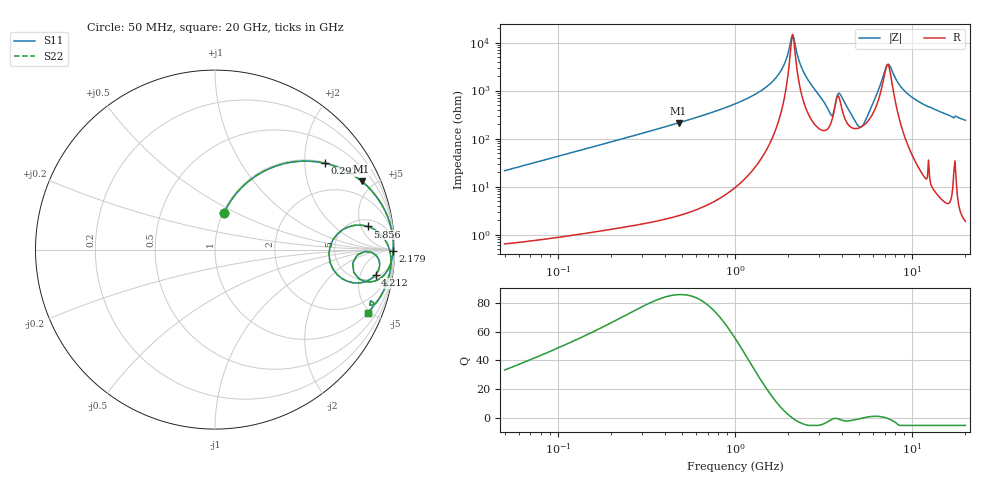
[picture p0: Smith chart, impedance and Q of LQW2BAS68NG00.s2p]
!Murata Part Number: LQW2BAS68NG00
!These Parameters are Measured in Series Mode Connection
!  o--[Z]--o
!Port1  Port2
!  o-------o
!Freq. Start=50[MHz] Stop=20[GHz], 401[Steps]
# Hz S RI R 50
!Freq.(Hz) S11(Real) S11(Imag) S21(Real) S21(Imag) S12(Real) S12(Imag) S22(Real) S22(Imag)
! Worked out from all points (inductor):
!   401 points, 50 MHz to 20 GHz, reference 50 ohm
!   read as one part in series: L = 68.3 nH near 51.52 MHz
!   highest Q = 85.5 at 480 MHz (marker M1), where L = 70.6 nH
!   self-resonance near 2.115 GHz
!   S11 on the Smith chart (normalised r, x): 50 MHz: 1.01, +0.43; 292.8 MHz: 1.03, +2.53; 2.179 GHz: open; 4.212 GHz: 6, -9; 5.856 GHz: 6.67, +6.62; 20 GHz: 1.04, -4.82
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5e7  0.0498 0.2031  0.9502 -0.2031  0.9502 -0.2031  0.0498 0.2031
1.364002e8  0.258 0.4287  0.742 -0.4287  0.742 -0.4287  0.258 0.4287
2.928045e8  0.6135 0.4805  0.3865 -0.4805  0.3865 -0.4805  0.6135 0.4805
3.721004e8  0.722 0.442  0.278 -0.442  0.278 -0.442  0.722 0.442
4.800071e8  0.8164 0.3813  0.1836 -0.3813  0.1836 -0.3813  0.8164 0.3813
1e9  0.9624 0.1814  0.0376 -0.1814  0.0376 -0.1814  0.9624 0.1814
1.639343e9  0.9917 0.0622  0.00833 -0.0622  0.00833 -0.0622  0.9917 0.0622
1.875929e9  0.9937 0.0302  0.00628 -0.0302  0.00628 -0.0302  0.9937 0.0302
2.083303e9  0.9935 0.00426  0.00654 -0.00426  0.00654 -0.00426  0.9935 0.00426
2.179053e9  0.9927 -0.00737  0.00726 0.00737  0.00726 0.00737  0.9927 -0.00737
2.383959e9  0.9899 -0.0321  0.0101 0.0321  0.0101 0.0321  0.9899 -0.0321
2.728004e9  0.9793 -0.076  0.0207 0.076  0.0207 0.076  0.9793 -0.076
3.466789e9  0.8025 -0.1628  0.1975 0.1628  0.1975 0.1628  0.8025 -0.1628
3.850025e9  0.9086 -0.0475  0.0914 0.0475  0.0914 0.0475  0.9086 -0.0475
4.212059e9  0.8949 -0.1404  0.1051 0.1404  0.1051 0.1404  0.8949 -0.1404
5.041459e9  0.6407 -0.0701  0.3593 0.0701  0.3593 0.0701  0.6407 -0.0701
5.856089e9  0.8506 0.1291  0.1494 -0.1291  0.1494 -0.1291  0.8506 0.1291
7.114996e9  0.969 0.0087  0.031 -0.0087  0.031 -0.0087  0.969 0.0087
7.442007e9  0.9753 -0.0144  0.0247 0.0144  0.0247 0.0144  0.9753 -0.0144
8.644534e9  0.9802 -0.0794  0.0198 0.0794  0.0198 0.0794  0.9802 -0.0794
1.019291e10  0.9718 -0.1394  0.0282 0.1394  0.0282 0.1394  0.9718 -0.1394
2e10  0.8512 -0.352  0.1488 0.352  0.1488 0.352  0.8512 -0.352
